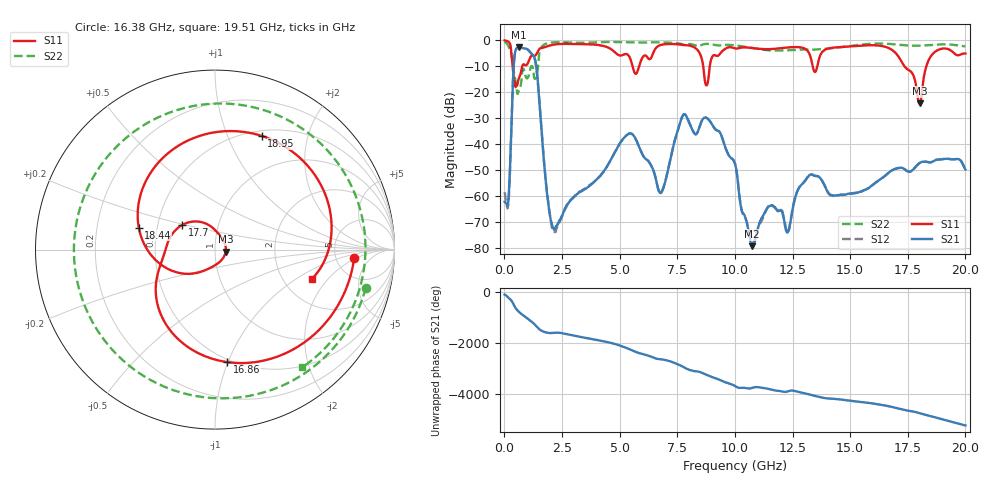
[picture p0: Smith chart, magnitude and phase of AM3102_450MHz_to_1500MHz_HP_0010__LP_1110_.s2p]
!Agilent Technologies,E8364B,MY43040894,A.07.50.67
!Agilent E8364B: A.07.50.67
!Date: Thursday, January 11, 2018 05:29:10
!Correction: S11(Full 2 Port(1,2))
!S21(Full 2 Port(1,2))
!S12(Full 2 Port(1,2))
!S22(Full 2 Port(1,2))
!S2P File: Measurements: S11, S21, S12, S22:
# Hz S  dB  R 50
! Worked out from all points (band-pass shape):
!   1601 points, 10 MHz to 20 GHz, reference 50 ohm
!   highest |S21| = -2.74 dB at 634.7 MHz (marker M1); lowest = -79.4 dB at 10.75 GHz (marker M2)
!   |S21| within 3 dB of the highest: 445.9 MHz to 1.243 GHz (796.7 MHz wide, 94.4 % of centre)
!   lowest |S11| = -24.3 dB at 18.01 GHz (marker M3), VSWR 1.13, Z = 56.3 - j1.28 ohm
!   |S11| at or under -10 dB: 357.8 MHz to 774.5 MHz (416.7 MHz wide, 73.6 % of centre); 5.559 GHz to 5.846 GHz (286.6 MHz wide, 5.03 % of centre); 17.36 GHz to 18.31 GHz (950.4 MHz wide, 5.33 % of centre)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
!   |S22| runs from -20.7 to -0.6 dB; largest |S21 - S12| = 0.0018
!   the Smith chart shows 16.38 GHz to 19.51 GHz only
!   S11 on the Smith chart (normalised r, x): 16.38 GHz: 7.50, -1.83; 16.86 GHz: 0.48, -0.99; 17.7 GHz: 0.67, +0.19; 18.44 GHz: 0.39, +0.12; 18.95 GHz: 0.56, +1.34; 19.51 GHz: 2.86, -1.38
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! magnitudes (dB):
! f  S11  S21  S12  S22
! 10 MHz  -0.1  -62.2  -58.5  -0.6
! 172.4 MHz  -0.6  -62.0  -62.8  -2.2
! 634.7 MHz  -14.6  -2.7  -2.7  -19.3
! 1.347 GHz  -5.8  -8.2  -8.2  -14.7
! 2.121 GHz  -1.7  -72.4  -73.4  -0.8
! 3.346 GHz  -1.5  -58.2  -57.9  -1.0
! 5.445 GHz  -6.7  -35.9  -35.9  -0.8
! 6.682 GHz  -2.2  -57.6  -57.6  -0.8
! 7.794 GHz  -1.8  -28.5  -28.5  -1.6
! 8.768 GHz  -17.4  -29.9  -29.9  -1.4
! 10.01 GHz  -3.1  -47.6  -47.6  -1.9
! 10.75 GHz  -3.0  -79.4  -78.3  -2.9
! 13.34 GHz  -8.5  -51.8  -51.7  -3.6
! 16.38 GHz  -2.2  -53.1  -53.2  -1.2
! 16.68 GHz  -3.0  -51.0  -50.9  -1.4
! 16.86 GHz  -4.0  -49.9  -49.9  -1.5
! 17.7 GHz  -12.8  -50.1  -50.1  -2.1
! 18.01 GHz  -24.3  -47.3  -47.3  -2.1
! 18.44 GHz  -7.1  -47.1  -47.1  -1.8
! 18.95 GHz  -3.3  -45.9  -45.8  -1.5
! 19.51 GHz  -5.0  -45.9  -45.9  -1.8
! 20 GHz  -5.1  -49.8  -49.8  -2.3
